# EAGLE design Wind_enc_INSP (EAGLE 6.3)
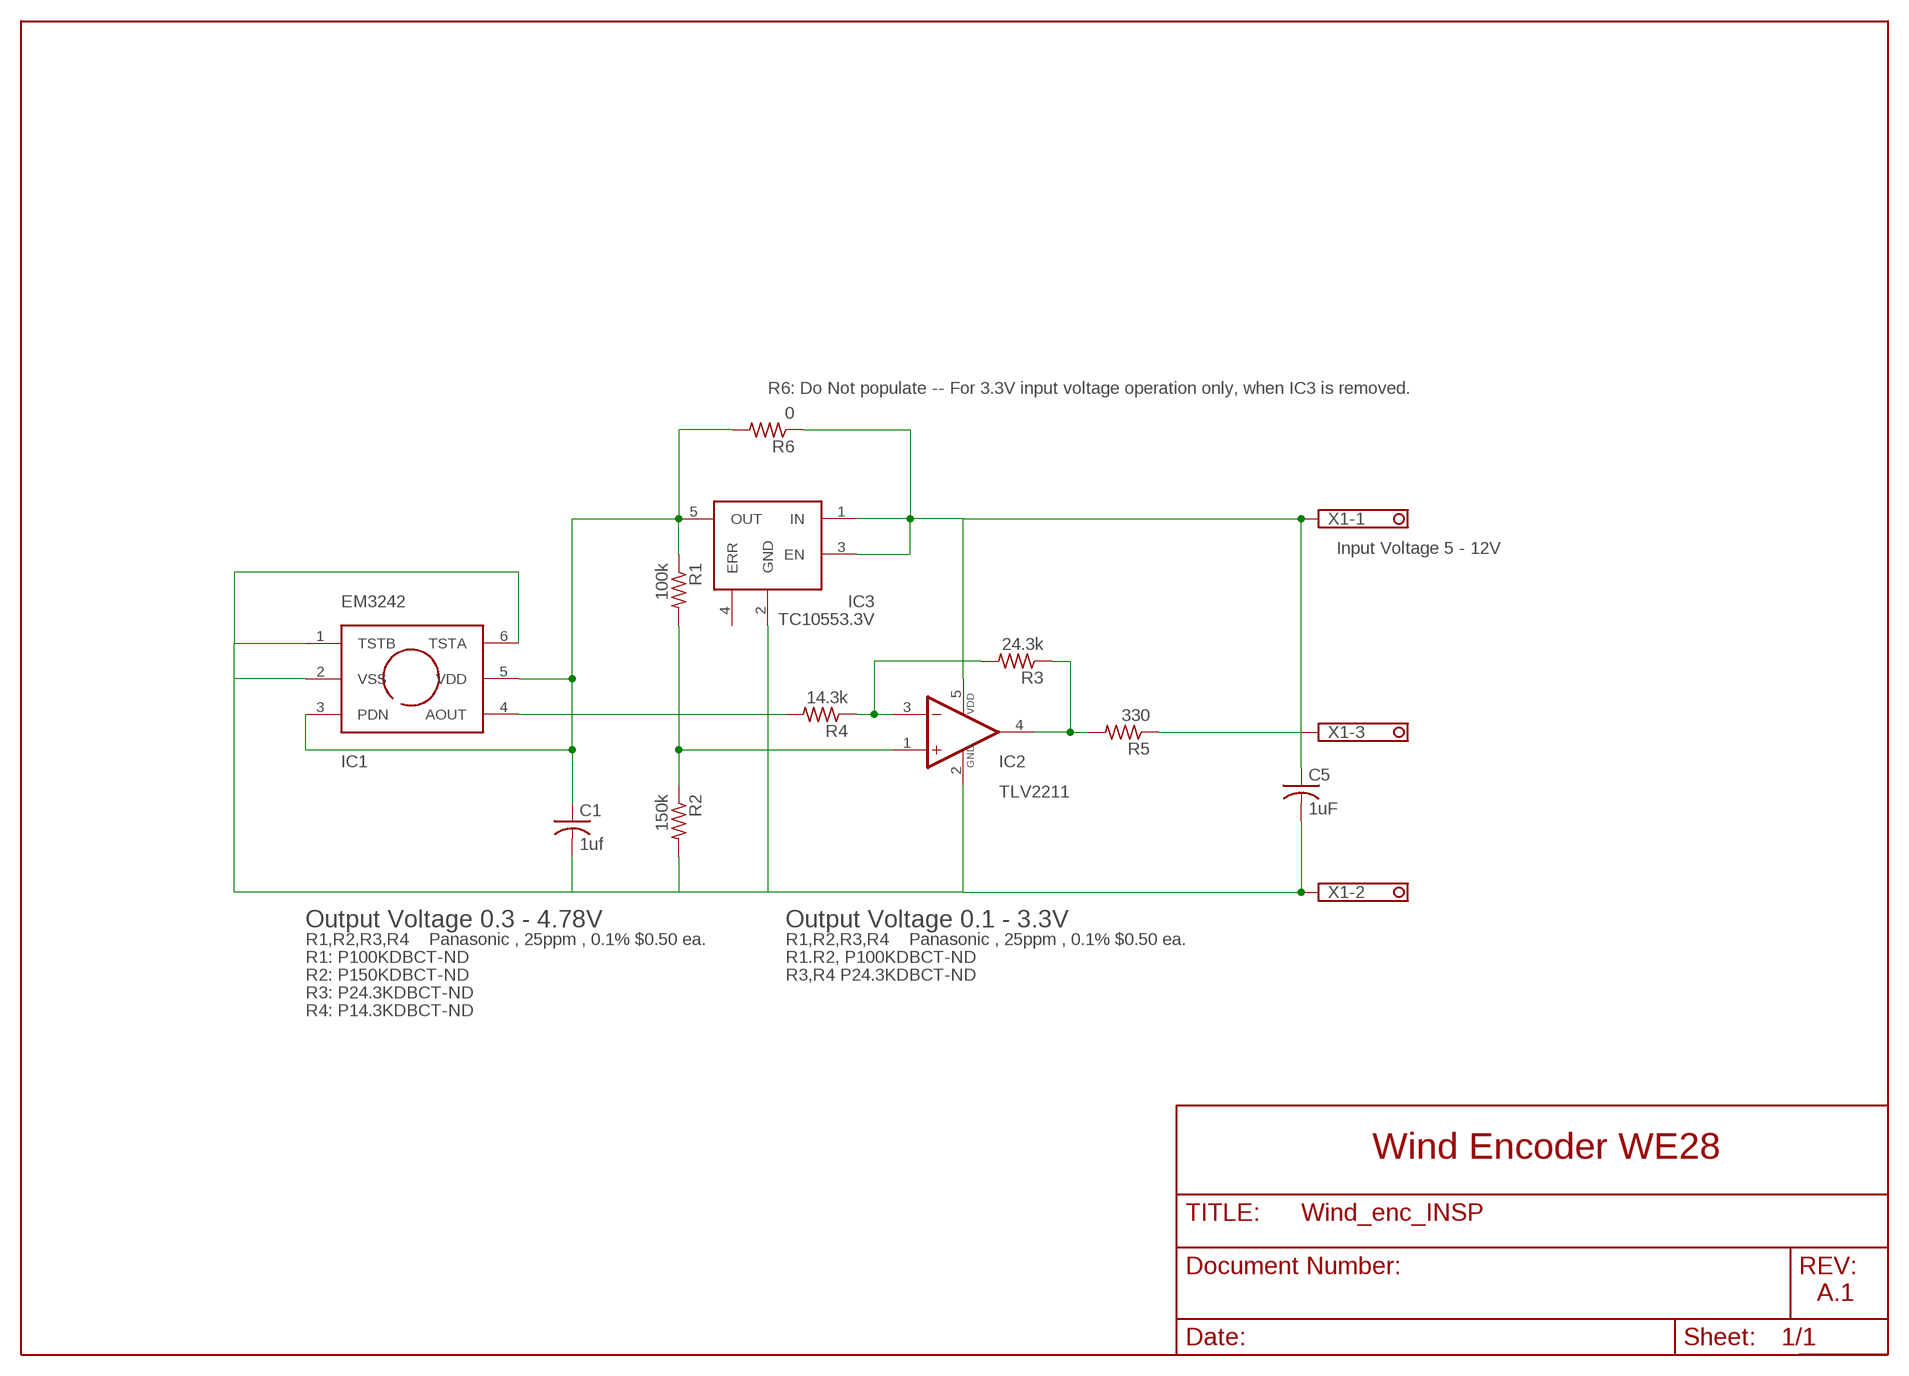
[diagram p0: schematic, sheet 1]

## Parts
C1  1uf  C-USC0805K  [C0805K]
C5  1uF  C-USC0805K  [C0805K]
IC1  EM3242  [EM3242_SPECIAL]
IC2  TLV2211  TLVB2211  [SOT23-5]
IC3  TC10553.3V  [SOT23-5]
R1  100k  R-US_R0603  [R0603]
R2  150k  R-US_R0603  [R0603]
R3  24.3k  R-US_R0603  [R0603]
R4  14.3k  R-US_R0603  [R0603]
R5  330  R-US_R0603  [R0603]
R6  0  R-US_R0603  [R0603]
X1  1751251  [1751251]

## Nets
N$1: C5.1 IC2.5(VDD) IC3.1(IN) IC3.3(EN) R6.1 X1.1
N$2: C1.2 C5.2 IC1.1(TSTB) IC1.2(VSS) IC1.6(TSTA) IC2.2(VDD_GND) IC3.2(GND) R2.2 X1.2
N$3: R5.1 X1.3
N$4: IC1.4(AOUT) R4.2
N$5: C1.1 IC1.3(PDN) IC1.5(VDD) IC3.5(OUT) R1.1 R6.2
N$6: IC2.3(-IN) R3.2 R4.1
N$7: IC2.4(OUT) R3.1 R5.2
N$8: IC2.1(+IN) R1.2 R2.1
Unconnected: IC3.4(ERR)

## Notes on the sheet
- R6: Do Not populate -- For 3.3V input voltage operation only, when IC3 is removed.
- Input Voltage 5 - 12V
- IC2
- Output Voltage 0.3 - 4.78V | Output Voltage 0.1 - 3.3V
- R1,R2,R3,R4    Panasonic , 25ppm , 0.1% $0.50 ea. | R1,R2,R3,R4    Panasonic , 25ppm , 0.1% $0.50 ea.
- R1: P100KDBCT-ND | R1.R2, P100KDBCT-ND
- R2: P150KDBCT-ND | R3,R4 P24.3KDBCT-ND
- R3: P24.3KDBCT-ND
- R4: P14.3KDBCT-ND
- Wind Encoder WE28
- A.1

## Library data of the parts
C1 C5 = rcl:C-US: CAPACITOR, American symbol
IC1 = 1AA_Stofer:EM3242: AsahiKasei single chip hall effect rotary encoder with DC out
IC2 = 1AA_Stofer:TLVB2211: TI Rail to Rail LINCMOS op-amp
IC3 = 1AA_Stofer:TC10553.3V
R1-R6 = rcl:R-US_: RESISTOR, American symbol
X1 = con-phoenix-350:1751251: MKDS 1/ 3-3,5 Printklemme Nennstrom: 10 A Bemessungsspannung: 160 V Raster: 3,5 mm Polzahl: 3 Montageart: Löten Anschlussart: Schraubanschluss Anschlussrichtung vom Leiter zur Platine: 0° Source: http://eshop.phoenixcontact.com .. 1751251.pdf; OC_FARNELL: unknown; OC_NEWARK: unknown

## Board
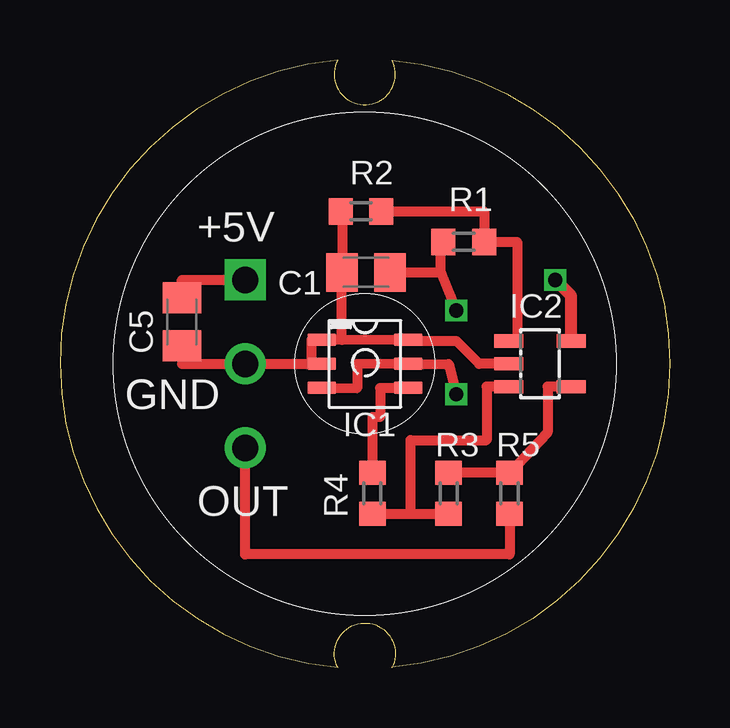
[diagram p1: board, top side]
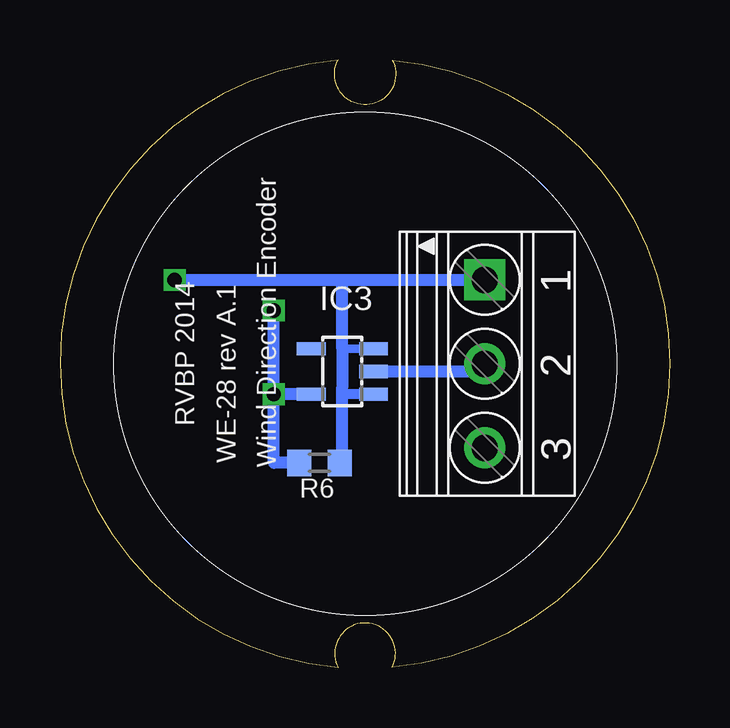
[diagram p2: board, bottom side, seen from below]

Size 25.41 x 25.32 mm. Coordinates in mm from the lower left corner, seen from the top.
Outline: 11.57,25.32 arc170 11.58,0.02
Outline: 11.57,25.32 arc235 13.83,25.32
Outline: 13.83,25.32 arc-170 13.82,0.01
Outline: 11.57,0.02 arc-235 13.83,0
Copper layers (1*16): Top 0.035mm / dielectric 1.5mm / Bottom 0.035mm
Design rules "Elecrow_2-layer_eagle_rule": minimum track width 6mil, minimum drill 12mil, track to track 6mil, track to pad 6mil, pad to pad 6mil, via to via 6mil, smd to smd 0mil, copper to edge 10mil, drill to drill 10mil, minimum pad ring 10mil, minimum via ring 6mil, stop-mask expansion 2mil, vias tented up to drill 100mil, thermal gap 10mil

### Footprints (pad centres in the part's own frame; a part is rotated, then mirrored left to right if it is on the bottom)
C0805K = smd 1.3 x 1.6: 1 -1,0; 2 1,0
EM3242_SPECIAL = smd 1.194 x 0.533: 1 -0.3,2; 2 -0.3,1; 3 -0.3,0; 4 3.3,0; 5 3.3,1; 6 3.3,2
SOT23-5 = smd 0.55 x 1.2: 1 -0.95,-1.3; 2 0,-1.3; 3 0.95,-1.3; 4 0.95,1.3; 5 -0.95,1.3
R0603 = smd 1 x 1.1: 1 -0.85,0; 2 0.85,0
1751251 = drill 1.1 pad 1.7 square: 1 -3.5,-0.1 | drill 1.1 pad 1.7: 2 0,-0.1; 3 3.5,-0.1

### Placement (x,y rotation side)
C1  12.75,16.47 180 top
C5  5.08,14.41 270 top
IC1  11.2,11.66 0 top
IC2  20,12.66 270 top
IC3  13.65,12.35 90 bottom
R1  16.83,17.74 0 top
R2  12.54,19.01 180 top
R3  16.19,7.27 270 top
R4  13.02,7.27 90 top
R5  18.73,7.27 90 top
R6  14.6,8.54 180 bottom
X1  7.62,12.66 270 bottom

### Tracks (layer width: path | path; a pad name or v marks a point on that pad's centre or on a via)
N$1  (via drill 0.6)
  Top 0.356: X1.1
  Top 0.406: C5.1 5.08,16.16 X1.1
  Top 0.508: IC2.5 21.3,15.49 v20.64,16.16
  Bottom 0.356: IC3.3 13.65,13.3 | 13.65,11.71 13.65,11.4 | X1.1
  Bottom 0.406: IC3.1 13.65,11.4 | R6.1 13.65,8.54
  Bottom 0.508: v20.64,16.16 13.65,16.16 | 13.65,16.16 X1.1 | 13.65,16.16 13.65,13.3 13.65,11.71 13.65,8.54
N$2
  Top 0.305: 14.51,13.62 IC1.6
  Top 0.356: 7.72,12.65 X1.2 | 11.69,16.26 11.75,16.26 C1.2 11.7,16.47 | 5.08,12.65 C5.2 | R2.2 11.75,19.01
  Top 0.406: IC1.2 10.48,12.65 | IC2.2 17.46,12.66 16.51,13.62 14.51,13.62 | 10.48,12.65 10.48,13.65 IC1.1 11.75,13.65 | IC1.6 11.75,13.65 | 11.75,13.65 11.75,16.26 | 10.48,12.65 7.72,12.65 5.08,12.65 | 11.75,19.01 C1.2
  Bottom 0.508: IC3.2 8.04,12.35 X1.2
N$3
  Top 0.406: R5.1 18.73,4.73 7.72,4.73 X1.3
N$4
  Top 0.254: IC1.4 14.29,11.65
  Top 0.406: 14.29,11.65 13.33,11.65 13.33,10.44 13.02,10.44 R4.2
N$5  (via drill 0.6)
  Top 0.406: IC1.3 12.38,11.65 12.38,12.65 IC1.5 16.19,12.65 v16.51,11.39 | C1.1 15.87,16.47 | 15.87,16.47 v16.51,14.89 | 15.87,16.47 15.87,17.64 R1.1
  Bottom 0.356: IC3.5
  Bottom 0.508: v16.51,11.39 v16.51,14.89 | IC3.5 v16.51,11.4 v16.51,11.39 | R6.2 16.51,8.54 v16.51,11.39
N$6
  Top 0.406: R4.1 14.6,6.42 | 14.6,6.42 R3.2 | 14.6,6.42 14.6,9.49 17.78,9.49 17.78,11.71 IC2.3
N$7
  Top 0.406: 16.51,8.12 R3.1 R5.2 20.32,9.81 20.32,11.71 IC2.4
N$8
  Top 0.356: IC2.1
  Top 0.406: IC2.1 19.05,13.62 19.05,17.74 R1.2 17.68,19.01 R2.1

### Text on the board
tPlace: +5V | GND | OUT
bPlace: Wind Direction Encoder | RVBP 2014 | WE-28 rev A.1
